//FC656	Send/Receive Schnittstelle - Ersatzwerte
// ***************************************************************************
FUNCTION "FC_SR_ERSA" : VOID

TITLE =Send/Receive Empfang

AUTHOR: 	SIEMENS
FAMILY: 	SISTARS7
VERSION: 	4.02

//KNOW_HOW_PROTECT

//Hinweis:


// Datum	 Name			Aktion
// ---------------------------------------------------------------------------
// 19.05.99  Mahler		Neu



//Eingabeparameter
VAR_INPUT
	iFKT			: INT;		//Aufrufmodus
	iVBNR			: INT;		//
END_VAR

//Ausgabeparameter
//VAR_OUTPUT
//END_VAR


//Temporäre/Lokale Variable
VAR_TEMP

	anyQUEL	: ANY; 	         //Offset=0, Zeiger muss an erster Stelle stehen
	anyZIEL	: ANY;		   //Offset=10,
	uVerb		:"XC_INIT_SR_UDT";   //Offset=20
	uJob		:"XC_JOB_SR_UDT";    //Offset=70


      iLoop		: INT;
//	iAct		: INT;

//	bCSend	: Byte;
//	bCRecv	: Byte;
//	bCSave	: Byte;

      dwPTR1	: DWORD;
      dwPTR2	: DWORD;

     	bTyp		: Byte;
	iDB		: INT;
	iDW		: INT;
	iAnz		: INT;
	iDBZ		: INT;
	iDWZ		: INT;

      bPCU		: Byte;

//   iRecvDW     : INT;

     iSysJob     : INT;
//   iDone		: INT;

	dwAR1		: DWORD;
      boERROR	: Bool;


END_VAR

BEGIN

NETWORK
TITLE = AR1 retten
// ===========================================================================

	TAR1	#dwAR1;


NETWORK
TITLE = Vorbesetzen der Zeiger
// ===========================================================================
//Pionter fuer den Empfangspuffer zusammenstellen
//Any-Pointer:
//Byte 0	: S7-Typ 		= 16=10H                 LB0,LB10
//Byte 1	: Datentyp		= 02=Byte			 LB1,LB11
//Byte 2/3	: Wiederholungsfaktor				 LW2,LW12
//Byte 4/5	: DB-Nummer						 LW4,LW14
//Byte 6-9	: Bereichszeiger					 LD6,LD16

	L 16;		//S7-Typ
	T LB 0;
	T LB 10;
	L 2;		//Datentyp=Byte
	T LB1;
	T LB11;



NETWORK
TITLE =Verbindungsfehler in den Job uebernehmen
// ===========================================================================
	L iFKT;
	L 1;
	<>I;
	spb end2;

	L   #iVBNR;
	+  -1;
	L   "XC_VERB_SR".iLen;
      *I;
	L   "XC_VERB_SR".iOffset;
	+I;
	SLD 3;
	lar1;
      t #dwPtr1;

      AUF   "XC_VERB_SR";
      U   DBX[AR1,p#0.7];         //Fehler
      =   #boERROR;

	L DBB[AR1,p#1.0];		//PCU-Nummer
      t #bPCU;


      l  1;				//Alle Jobs in einer Schleife untersuchen
	t #iSysJob;


Lo24:	L   #iSysJob;			//Schleifenanfang  1 ...256 Anwenderjobs untersuchen
	+  -1;
	L   "XC_JOB_SR".iLen;
      *I;
	L   "XC_JOB_SR".iOffset;      //Offset zu den Anwenderjobs
	+I;
	SLD 3;
	LAR1;			//Bereichszeiger

	auf "XC_JOB_SR";
      l DBW[AR1,p#0.0];       //PCU-Nummer
      l #bPCU;
      <>I;
	spb ne20;

      U   #boERROR;         //Fehler
      = DBX [AR1,P#3.2];      //Fehler in der PCU-Verbindung

ne20: l #iSysJob;
	l 1;
	+I;
      t #iSysJob;
	L  "XC_JOB_SR".iAct;
	<=I;
	spb Lo24;



end2: nop 0;


NETWORK
TITLE =Zyklischer Teil:  FKT 2 - Ersatzwerte umladen
// ===========================================================================

	l #iFkt;
	l 2;
	<>I;
      spb end4;

      l  1;				//Alle Jobs in einer Schleife untersuchen
	t #iSysJob;


Lo44:	L   #iSysJob;			//Schleifenanfang 1 ... 256 Anwenderjobs
	+  -1;
	L   "XC_JOB_SR".iLen;
      *I;
	L   "XC_JOB_SR".iOffset;      //Offset zu den Anwenderjobs
	+I;
	SLD 3;
	T #dwPTR1;		//Bereichszeiger

	LAR1 p#70.0;       //Pionter auf uVERB in den lokalen Daten
	auf  "XC_JOB_SR";

//Schleife um Daten in lokale Variable Byteweise umzuladen
	L  "XC_JOB_SR".iLen;		//Anzahl der Bytes
Lo45: T #iLoop;

      L DBB[#dwPTR1];		//Wert aus DB holen
	T LB [AR1,p#0.0];		//Wert in uVERB eintragen

	+AR1 p#1.0;			//AR1 um 1Bytes erhoehen
	l  #dwPTR1;			//Zeiger fuer DB-Datenwort erhoehen
	L 8;
	+D;
	T #dwPTR1;
	L   #iLoop;			//Schleifenzaehler erniedrigen und zum Anfang
	LOOP Lo45;

      L  #uJob.bFltSrc_AREA;  //Pruefen ob Ersatzwerte da
      L 0;
	==I;
	spb ne40;
	l #uJob.iFltTime;        //Sollzeit
      l #uJob.iFltActTime ;    //Istzeit
      <>I;
	spb ne40;
 	l #uJob.iFltActTime;     //Istzeit erhoehen um Bearbeitung der
      l 1;				 //Ersatzwerte wieder zu sperren
	+I;
 	t #uJob.iFltActTime;

     l #uJob.iFltSrc_DB;   //Quell DB
     t #iDB;
     l #uJob.dwFltSrcByte; //Quell Byte
     t #iDW;
     l #uJob.iFltSrc_Num;  //Anzahl
     t #iAnz;
     l #uJob.iDest_DB;   //Ziel DB
     t #iDBZ;
     l #uJob.dwDestByte; //Ziel Byte
     t #iDWZ;


     call "FC_COPY" (
                      iQDB	:=#iDB,
			    iQDW	:=#iDW,
                      bQTyp   :=B#16#84,
			    iZDB	:=#iDBZ,
		          iZDW	:=#iDWZ,
	                bZTyp   :=B#16#84,
			    iLenByte:=#iAnz
			    );




  	l  #iSysJob;			//Job wieder zurueck
	+  -1;
	L   "XC_JOB_SR".iLen;
      *I;
	L   "XC_JOB_SR".iOffset;
	+I;
	SLD 3;
	T #dwPTR1;		//Bereichszeiger

	LAR1 p#70.0;       //Pionter auf uVERB in den lokalen Daten
	auf  "XC_JOB_SR";

//Schleife um Daten in lokale Variable Byteweise umzuladen
	L  "XC_JOB_SR".iLen;		//Anzahl der Bytes
Lo46: T #iLoop;

    	L LB [AR1,p#0.0];		//Wert in uVERB eintragen
	T DBB[#dwPTR1];		//Wert aus DB holen

	+AR1 p#1.0;			//AR1 um 1Bytes erhoehen
	l  #dwPTR1;			//Zeiger fuer DB-Datenwort erhoehen
	L 8;
	+D;
	T #dwPTR1;
	L   #iLoop;			//Schleifenzaehler erniedrigen und zum Anfang
	LOOP Lo46;

ne40: l #iSysJob;
	l 1;
	+I;
      t #iSysJob;
	L  "XC_JOB_SR".iAct;
	<=I;
	spb Lo44;

end4: nop 0;


NETWORK
TITLE = AR1 zurück, ENDE
// ===========================================================================

	LAR1	#dwAR1;


END_FUNCTION
